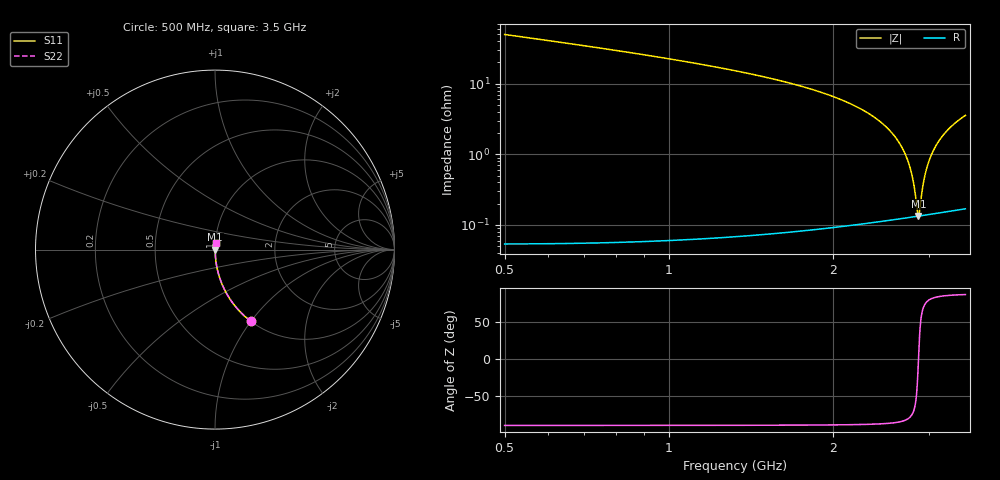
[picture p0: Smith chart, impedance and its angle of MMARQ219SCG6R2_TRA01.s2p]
! MMARQ219SCG6R2_TRA01  S-PARAMETER MODEL  ( General Type )
! Model Generated by TAIYO YUDEN Corporation (http://www.ty-top.com)
! Version 1.0
! TAIYO YUDEN Control No. 160201
! Copyright(c) 2016 TAIYO YUDEN CO.,LTD. All Rights Reserved.
! Product Description (link to TY-COMPAS)
! https://ds.yuden.co.jp/TYCOMPAS/or/detail?pn=MMARQ219SCG6R2CTRA01&u=M
! Products Name : Multilayer Ceramic Capacitors
! Characteristics :
!  Capacitance : 6.2 pF , Rated Voltage : 250V , TCC : CG / C0G
!  Case Size : 2.0 x 1.25 / 0.079 x 0.049 [mm/inch] , Thickness : 0.85 / 0.033 [mm/inch]
!  (Conditions: Temperature = 25 degC , DC Bias Current/Voltage = 0A / 0V)
! External Node Assignments :
!  1  o---| |---o  2
! GND o---------o GND
! Frequency Range : 500MHz  -  3500MHz  [ 401 STEP ]
# MHz S RI R 50
! Freq[MHz].  S11 Real  S11 Imag  S21 Real  S21 Imag  S12 Real  S12 Imag  S22 Real  S22 Imag
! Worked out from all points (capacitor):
!   401 points, 500 MHz to 3.5 GHz, reference 50 ohm
!   read as one part in series: C = 6.19 pF near 515 MHz
!   lowest |Z| = 133 mohm at 2.87 GHz (marker M1)
!   series resonance near 2.871 GHz, so ESL is about 500 pH
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500  0.1992 -0.3989  0.8008 0.3989  0.8008 0.3989  0.1992 -0.3989
710  0.1039 -0.3043  0.8961 0.3043  0.8961 0.3043  0.1039 -0.3043
1002.5  0.0487 -0.2139  0.9513 0.2139  0.9513 0.2139  0.0487 -0.2139
1505  0.0158 -0.1217  0.9842 0.1217  0.9842 0.1217  0.0158 -0.1217
2000  0.00525 -0.0656  0.9948 0.0656  0.9948 0.0656  0.00525 -0.0656
2292.5  0.00268 -0.0404  0.9973 0.0404  0.9973 0.0404  0.00268 -0.0404
2502.5  0.00175 -0.0245  0.9983 0.0245  0.9983 0.0245  0.00175 -0.0245
2645  0.00143 -0.0146  0.9986 0.0146  0.9986 0.0146  0.00143 -0.0146
2742.5  0.00133 -0.00816  0.9987 0.00816  0.9987 0.00816  0.00133 -0.00816
2772.5  0.00132 -0.00622  0.9987 0.00622  0.9987 0.00622  0.00132 -0.00622
2802.5  0.00131 -0.0043  0.9987 0.0043  0.9987 0.0043  0.00131 -0.0043
2825  0.00132 -0.00287  0.9987 0.00287  0.9987 0.00287  0.00132 -0.00287
2855  0.00132 -0.000992  0.9987 0.000992  0.9987 0.000992  0.00132 -0.000992
2870  0.00133 -5.92e-05  0.9987 5.92e-05  0.9987 5.92e-05  0.00133 -5.92e-05
2885  0.00134 0.000869  0.9987 -0.000869  0.9987 -0.000869  0.00134 0.000869
2922.5  0.00137 0.00317  0.9986 -0.00317  0.9986 -0.00317  0.00137 0.00317
2945  0.00139 0.00453  0.9986 -0.00453  0.9986 -0.00453  0.00139 0.00453
3005  0.00147 0.00813  0.9985 -0.00813  0.9985 -0.00813  0.00147 0.00813
3087.5  0.00162 0.013  0.9984 -0.013  0.9984 -0.013  0.00162 0.013
3192.5  0.00187 0.0189  0.9981 -0.0189  0.9981 -0.0189  0.00187 0.0189
3335  0.00231 0.0267  0.9977 -0.0267  0.9977 -0.0267  0.00231 0.0267
3500  0.00295 0.0354  0.9971 -0.0354  0.9971 -0.0354  0.00295 0.0354
